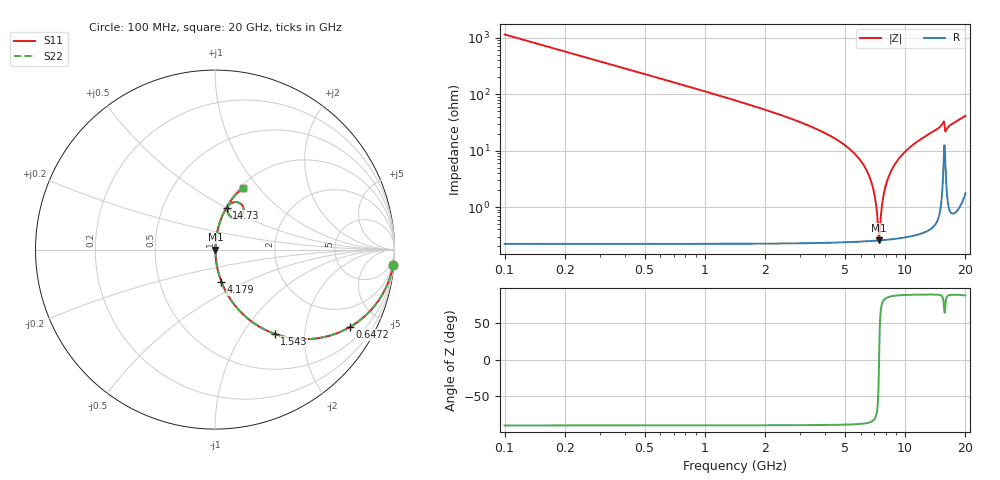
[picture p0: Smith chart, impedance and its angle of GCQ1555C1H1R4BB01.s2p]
!Murata Part Number: GCQ1555C1H1R4BB01
!These Parameters are Measured in Series Mode Connection
!Data Generated on Mar 13, 2026
!  o--ll--o
!Port1  Port2
!  o------o
!Operation Temp=25[degC], DC Bias Voltage=0[V]
!Freq. Start=100[MHz] Stop=20[GHz] 401[Steps]
# Hz S RI R 50
!Freq.(Hz) S11(Real) S11(Imag) S21(Real) S21(Imag) S12(Real) S12(Imag) S22(Real) S22(Imag)
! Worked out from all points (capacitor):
!   401 points, 100 MHz to 20 GHz, reference 50 ohm
!   read as one part in series: C = 1.4 pF near 199.5 MHz
!   lowest |Z| = 256 mohm at 7.413 GHz (marker M1)
!   series resonance near 7.412 GHz, so ESL is about 330 pH
!   S11 on the Smith chart (normalised r, x): 100 MHz: 1, -23; 647.2 MHz: 1.00, -3.49; 1.543 GHz: 1.00, -1.41; 4.179 GHz: 1.00, -0.37; 14.73 GHz: 1.01, +0.50; 20 GHz: 1.03, +0.82
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1e8  0.9923 -0.0873  0.0077 0.0873  0.0077 0.0873  0.9923 -0.0873
3.4875e8  0.9135 -0.2808  0.0865 0.2808  0.0865 0.2808  0.9135 -0.2808
6.4725e8  0.7521 -0.4312  0.2479 0.4312  0.2479 0.4312  0.7521 -0.4312
1.54275e9  0.3327 -0.4696  0.6673 0.4696  0.6673 0.4696  0.3327 -0.4696
2.33875e9  0.1623 -0.3662  0.8377 0.3662  0.8377 0.3662  0.1623 -0.3662
3.43325e9  0.0655 -0.243  0.9345 0.243  0.9345 0.243  0.0655 -0.243
4.1795e9  0.0356 -0.1791  0.9644 0.1791  0.9644 0.1791  0.0356 -0.1791
5.82125e9  0.00802 -0.0745  0.992 0.0745  0.992 0.0745  0.00802 -0.0745
6.7665e9  0.00329 -0.0281  0.9967 0.0281  0.9967 0.0281  0.00329 -0.0281
7.065e9  0.00274 -0.0148  0.9973 0.0148  0.9973 0.0148  0.00274 -0.0148
7.31375e9  0.00256 -0.00412  0.9974 0.00412  0.9974 0.00412  0.00256 -0.00412
7.41325e9  0.00255 5.16e-05  0.9974 -5.16e-05  0.9974 -5.16e-05  0.00255 5.16e-05
7.7615e9  0.00279 0.0142  0.9972 -0.0142  0.9972 -0.0142  0.00279 0.0142
8.20925e9  0.00364 0.0316  0.9964 -0.0316  0.9964 -0.0316  0.00364 0.0316
8.9555e9  0.00621 0.0588  0.9938 -0.0588  0.9938 -0.0588  0.00621 0.0588
1.005e10  0.0121 0.0956  0.9879 -0.0956  0.9879 -0.0956  0.0121 0.0956
1.338325e10  0.0432 0.1937  0.9568 -0.1937  0.9568 -0.1937  0.0432 0.1937
1.47265e10  0.0654 0.2343  0.9346 -0.2343  0.9346 -0.2343  0.0654 0.2343
1.557225e10  0.1379 0.2592  0.8621 -0.2592  0.8621 -0.2592  0.1379 0.2592
1.59205e10  0.0844 0.1861  0.9156 -0.1861  0.9156 -0.1861  0.0844 0.1861
1.67165e10  0.0779 0.253  0.9221 -0.253  0.9221 -0.253  0.0779 0.253
2e10  0.1554 0.3417  0.8446 -0.3417  0.8446 -0.3417  0.1554 0.3417
